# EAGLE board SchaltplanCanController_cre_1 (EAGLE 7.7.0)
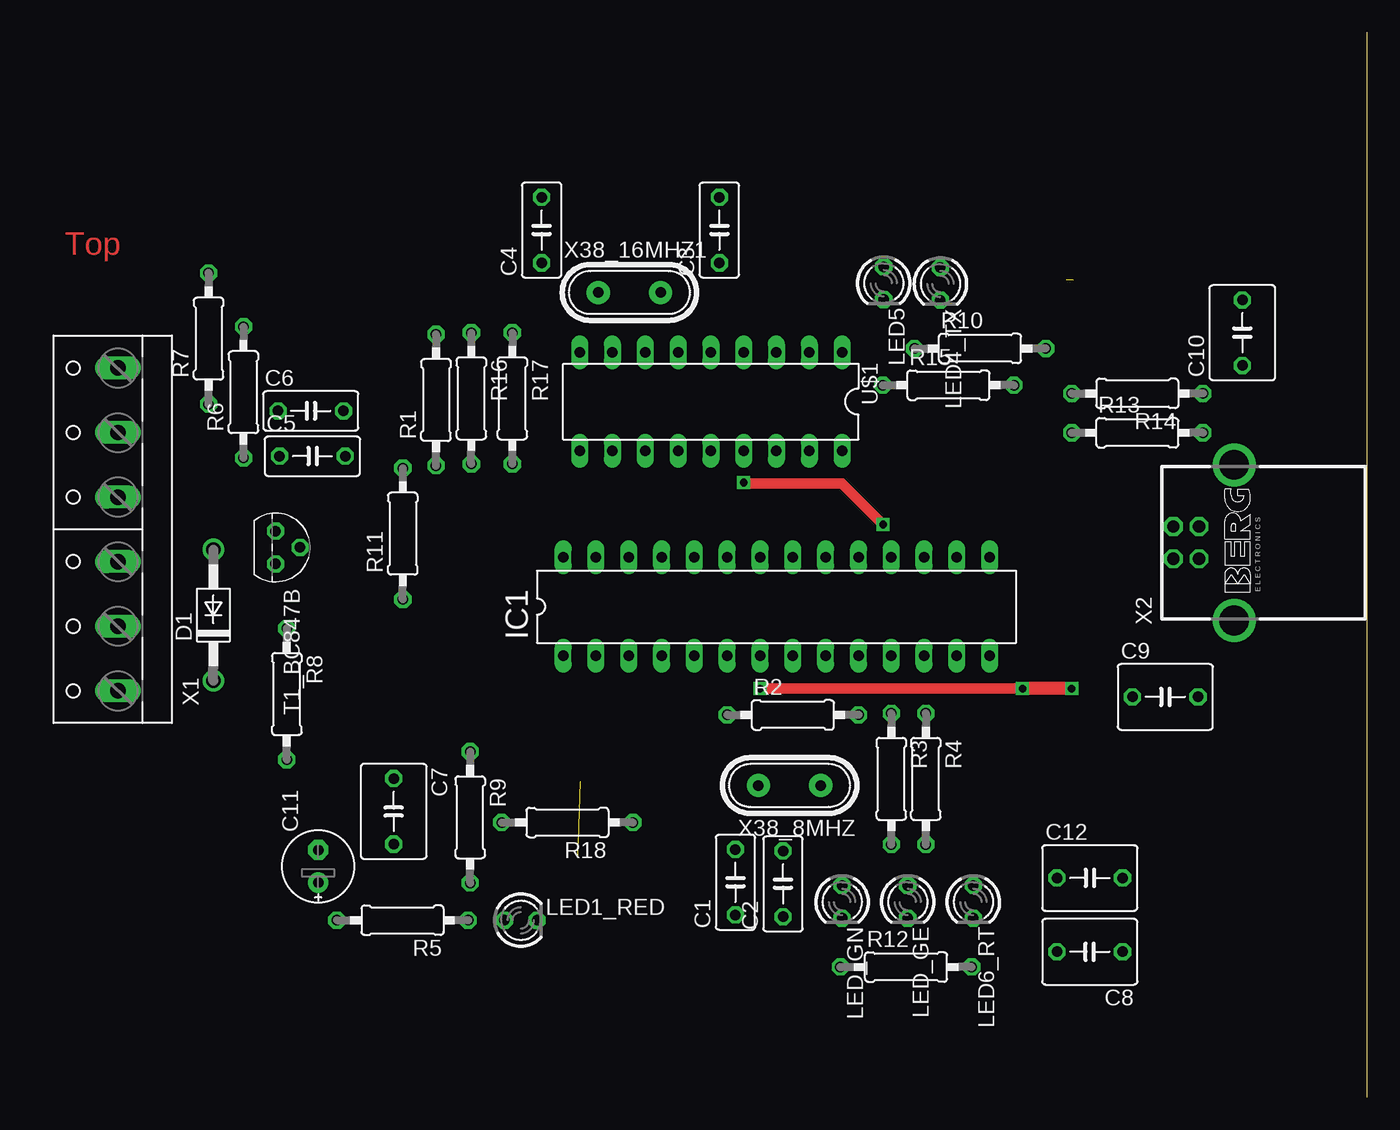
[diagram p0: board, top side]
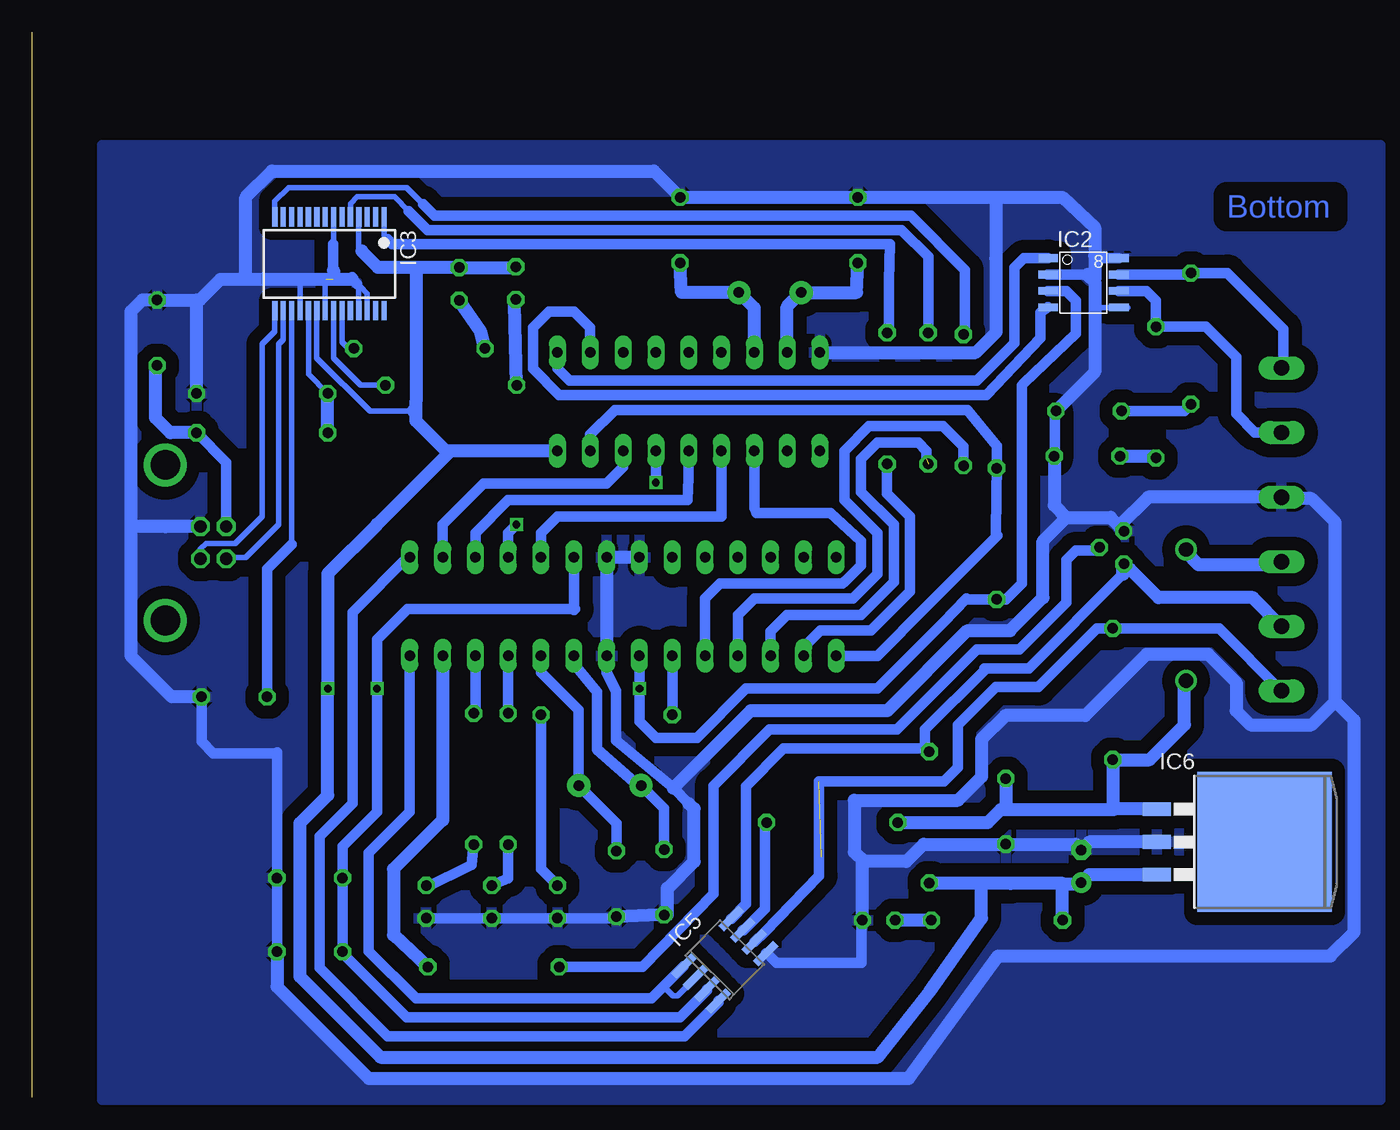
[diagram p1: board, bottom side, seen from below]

Size 0 x 82.46 mm. Coordinates in mm from the lower left corner, seen from the top.
Outline: 0,0 0,82.46
Copper layers (1*16): Top 0.035mm / dielectric 1.5mm / Bottom 0.035mm
Design rules "default": minimum track width 10mil, minimum drill 24mil, track to track 8mil, track to pad 8mil, pad to pad 8mil, via to via 8mil, smd to smd 8mil, copper to edge 40mil, drill to drill 8mil, minimum pad ring 10mil, minimum via ring 8mil, stop-mask expansion 4mil, vias tented up to drill 0mil, thermal gap 10mil

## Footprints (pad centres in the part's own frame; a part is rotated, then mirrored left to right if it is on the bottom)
C050-030X075 = drill 0.813 octagon: 1 -2.54,0; 2 2.54,0
C050-050X075 = drill 0.813 octagon: 1 -2.54,0; 2 2.54,0
E2,5-6E = drill 0.813 pad 1.575: + -1.27,0 | drill 0.813 pad 1.575 octagon: - 1.27,0
DO41-10 = drill 1.118: A 5.08,0; C -5.08,0
DIL28-3 = drill 0.813 long: 1 -16.51,-3.81; 2 -13.97,-3.81; 3 -11.43,-3.81; 4 -8.89,-3.81; 5 -6.35,-3.81; 6 -3.81,-3.81; 7 -1.27,-3.81; 8 1.27,-3.81; 9 3.81,-3.81; 10 6.35,-3.81; 11 8.89,-3.81; 12 11.43,-3.81; 13 13.97,-3.81; 14 16.51,-3.81; 15 16.51,3.81; 16 13.97,3.81; 17 11.43,3.81; 18 8.89,3.81; 19 6.35,3.81; 20 3.81,3.81; 21 1.27,3.81; 22 -1.27,3.81; 23 -3.81,3.81; 24 -6.35,3.81; 25 -8.89,3.81; 26 -11.43,3.81; 27 -13.97,3.81; 28 -16.51,3.81
DIL08 = smd 1.524 x 0.61: 1 -2.743,1.905; 2 -2.743,0.635; 3 -2.743,-0.635; 4 -2.743,-1.905; 5 2.743,-1.905; 6 2.743,-0.635; 7 2.743,0.635; 8 2.743,1.905
SSOP28 = smd 0.4 x 1.5: 1 -4.225,-3.625; 2 -3.575,-3.625; 3 -2.925,-3.625; 4 -2.275,-3.625; 5 -1.625,-3.625; 6 -0.975,-3.625; 7 -0.325,-3.625; 8 0.325,-3.625; 9 0.975,-3.625; 10 1.625,-3.625; 11 2.275,-3.625; 12 2.925,-3.625; 13 3.575,-3.625; 14 4.225,-3.625; 15 4.225,3.625; 16 3.575,3.625; 17 2.925,3.625; 18 2.275,3.625; 19 1.625,3.625; 20 0.975,3.625; 21 0.325,3.625; 22 -0.325,3.625; 23 -0.975,3.625; 24 -1.625,3.625; 25 -2.275,3.625; 26 -2.925,3.625; 27 -3.575,3.625; 28 -4.225,3.625
SO08 = smd 0.6 x 2.2: 1 -1.905,-2.6; 2 -0.635,-2.6; 3 0.635,-2.6; 4 1.905,-2.6; 5 1.905,2.6; 6 0.635,2.6; 7 -0.635,2.6; 8 -1.905,2.6
TO263-3 = smd 1.067 x 2.159: 1 -2.54,-5.791; 2 0,-5.791; 3 2.54,-5.791 | smd 10.8 x 10.41: TAB 0,2.54
LED3MM = drill 0.813 octagon: A -1.27,0; K 1.27,0
0207/10 = drill 0.813 octagon: 1 -5.08,0; 2 5.08,0
TO92 = drill 0.813 octagon: 1 1.27,0; 2 0,1.905; 3 -1.27,0
DIL18 = drill 0.813 long: 1 -10.16,-3.81; 2 -7.62,-3.81; 3 -5.08,-3.81; 4 -2.54,-3.81; 5 0,-3.81; 6 2.54,-3.81; 7 5.08,-3.81; 8 7.62,-3.81; 9 10.16,-3.81; 10 10.16,3.81; 11 7.62,3.81; 12 5.08,3.81; 13 2.54,3.81; 14 0,3.81; 15 -2.54,3.81; 16 -5.08,3.81; 17 -7.62,3.81; 18 -10.16,3.81
W237-6 = drill 1.194 long: 1 -12.5,-1.27; 2 -7.5,-1.27; 3 -2.5,-1.27; 4 2.5,-1.27; 5 7.5,-1.27; 6 12.5,-1.27
PN61729-S = drill 0.95 octagon: 1 1.25,4.71; 2 -1.25,4.71; 3 -1.25,2.71; 4 1.25,2.71 | drill 2.3 pad 2.9: S1 -6.02,0; S2 6.02,0
HC49 = drill 0.813 pad 1.8: 1 -2.413,0; 2 2.413,0

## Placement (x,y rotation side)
C1  22pF  [C050-030X075]  -48.91,16.65 90 top  (outside the outline)
C2  22pF  [C050-030X075]  -45.23,16.53 90 top  (outside the outline)
C3  22pF  [C050-030X075]  -50.16,67.15 90 top  (outside the outline)
C4  22pF  [C050-030X075]  -63.91,67.15 90 top  (outside the outline)
C5  560pF  [C050-030X075]  -81.66,49.64 0 top  (outside the outline)
C6  560pF  [C050-030X075]  -81.79,53.15 0 top  (outside the outline)
C7  100nF  [C050-050X075]  -75.37,22.14 270 top  (outside the outline)
C8  100nF  [C050-050X075]  -21.48,11.27 180 top  (outside the outline)
C9  100nF  [C050-050X075]  -15.64,31 0 top  (outside the outline)
C10  10nF  [C050-050X075]  -9.67,59.2 90 top  (outside the outline)
C11  10uf  [E2,5-6E]  -81.21,17.89 90 top  (outside the outline)
C12  100nF  [C050-050X075]  -21.48,16.98 0 top  (outside the outline)
D1  1N4004  [DO41-10]  -89.32,37.33 90 top  (outside the outline)
IC1  MEGA48/88/168-PU  [DIL28-3]  -45.73,37.99 0 top  (outside the outline)
IC2  SNOWND  [DIL08]  -81.38,63.07 0 bottom  (outside the outline)
IC3  FT232RL  [SSOP28]  -23,64.53 180 bottom  (outside the outline)
IC5  L9637D  [SO08]  -53.61,10.65 315 bottom  (outside the outline)
IC6  LM2937  [TO263-3]  -92.85,19.78 270 bottom  (outside the outline)
LED1_RED  2mA_+3,3V  [LED3MM]  -65.52,13.71 0 top  (outside the outline)
LED4_TX  2mA_TX  [LED3MM]  -33.04,62.98 270 top  (outside the outline)
LED5  2mA_RX  [LED3MM]  -37.43,63.03 270 top  (outside the outline)
LED6_RT  2mA mC  [LED3MM]  -30.49,15.13 270 top  (outside the outline)
LED_GE  2mA mC  [LED3MM]  -35.58,15.13 270 top  (outside the outline)
LED_GN  2mA mC  [LED3MM]  -40.65,15.13 270 top  (outside the outline)
R1  0  [0207/10]  -72.09,53.99 90 top  (outside the outline)
R2  270  [0207/10]  -44.46,29.61 0 top  (outside the outline)
R3  270  [0207/10]  -36.84,24.66 270 top  (outside the outline)
R4  270  [0207/10]  -34.18,24.66 270 top  (outside the outline)
R5  100  [0207/10]  -74.68,13.71 180 top  (outside the outline)
R6  100  [0207/10]  -87,54.59 90 top  (outside the outline)
R7  100  [0207/10]  -89.69,58.75 90 top  (outside the outline)
R8  510  [0207/10]  -83.64,31.22 270 top  (outside the outline)
R9  510  [0207/10]  -69.45,21.68 270 top  (outside the outline)
R10  270  [0207/10]  -29.97,57.98 0 top  (outside the outline)
R11  10k  [0207/10]  -74.66,43.64 90 top  (outside the outline)
R12  1k  [0207/10]  -35.7,10.09 0 top  (outside the outline)
R13  4k7  [0207/10]  -17.8,51.45 0 top  (outside the outline)
R14  10k  [0207/10]  -17.8,54.5 180 top  (outside the outline)
R15  270  [0207/10]  -32.42,55.13 0 top  (outside the outline)
R16  0  [0207/10]  -69.36,54.12 270 top  (outside the outline)
R17  0  [0207/10]  -66.18,54.12 270 top  (outside the outline)
R18  0  [0207/10]  -61.92,21.28 180 top  (outside the outline)
T1_BC847B  2N3565  [TO92]  -84.52,42.57 270 top  (outside the outline)
U$1  MCP2515DIL  [DIL18]  -50.81,53.87 180 top  (outside the outline)
X1  [W237-6]  -97.98,43.97 90 top  (outside the outline)
X2  PN61729-S  [PN61729-S]  -10.3,42.94 90 top  (outside the outline)
X38_8MHZ  CRYSTALS-NOGND-HC49  [HC49]  -44.72,24.15 180 top  (outside the outline)
X38_16MHZ1  CRYSTALS-NOGND-HC49  [HC49]  -57.12,62.31 0 top  (outside the outline)

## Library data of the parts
C1-C12 R1-R18 = rcl
D1 = diode
IC1 = avr-6
IC2 = SN65HVD231D
IC3 = ftdichip; MPN: FT232RL; OC_FARNELL: 1146032; OC_NEWARK: 91K9918
IC5 = st-microelectronics
IC6 = linear
LED1_RED LED4_TX LED5 LED6_RT LED_GE LED_GN = led
T1_BC847B = transistor
U$1 = MCP2515_MT
X1 = con-wago-500; OC_FARNELL: unknown; OC_NEWARK: unknown
X2 = con-berg; OC_FARNELL: unknown; OC_NEWARK: unknown
X38_8MHZ X38_16MHZ1 = IQD-Frequency-Products

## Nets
+5V: C8.2 C11.+ C12.1 IC1.7 IC1.20 IC2.3 IC3.4 IC3.20 IC5.3 IC6.3 LED4_TX.A LED5.A R5.2 R9.2 R11.1 U$1.18
+10V: C7.1 D1.C IC6.1 R8.2 R18.2
+12V: D1.A X1.3
GND: C1.1 C2.1 C3.2 C4.2 C5.2 C6.2 C7.2 C8.1 C9.2 C10.2 C11.- C12.2 IC1.8 IC1.21 IC1.22 IC2.2 IC2.8 IC3.7 IC3.18 IC3.21 IC3.25 IC3.26 IC5.5 IC6.2 LED1_RED.K LED6_RT.K LED_GE.K LED_GN.K R14.1 T1_BC847B.3 U$1.9 X1.4 X2.4
N$1: LED1_RED.A R5.1
N$2: IC1.1 R11.2 U$1.17
N$3: C1.2 IC1.9 X38_8MHZ.2
N$4: C5.1 R6.1
N$5: IC2.4 U$1.2
N$6: IC1.16 U$1.16
N$7: C2.2 IC1.10 X38_8MHZ.1
N$8: IC1.18 U$1.15
N$9: IC1.17 U$1.14
N$10: IC1.19 U$1.13
N$11: C3.1 U$1.7 X38_16MHZ1.2
N$12: C4.1 U$1.8 X38_16MHZ1.1
N$13: IC1.5 U$1.12
N$14: C6.1 R7.1
N$15: IC2.1 U$1.1
N$16: LED6_RT.A R4.2
N$17: IC1.14 IC5.1 IC5.2
N$18: IC1.15 IC5.4
N$19: IC3.16 X2.2
N$20: IC2.6 R6.2 X1.5
N$21: IC2.7 R7.2 X1.6
N$23: LED5.K R15.1
N$24: LED_GN.A R2.2
N$25: IC1.6 R2.1
N$26: IC1.11 R3.1
N$27: IC1.12 R4.1
N$28: LED_GE.A R3.2
N$29: IC3.15 X2.3
N$30: LED4_TX.K R10.1
N$31: IC1.2 R17.2
N$32: IC3.22 R15.2
N$33: IC5.6 R8.1 X1.1
N$34: R12.1 T1_BC847B.2
N$35: IC1.13 R12.2
N$36: IC5.8 R9.1 T1_BC847B.1 X1.2
N$37: C10.1 R13.2 X2.1
N$38: C9.1 IC3.17
N$39: IC3.23 R10.2
N$40: IC3.14 R1.2
N$41: IC1.4 R1.1
N$42: IC3.1 R17.1
N$43: IC5.7 R18.1
N$45: IC1.3 R16.2
N$46: IC3.5 R16.1
N$47: IC3.19 R13.1 R14.2

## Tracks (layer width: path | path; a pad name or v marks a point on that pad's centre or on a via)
+5V  (via drill 0.6)
  Top 0.813: v-47,31.64 v-26.69,31.64
  Top 1.016: v-22.88,31.64 v-26.69,31.64
  Bottom 0.406: IC3.4 -25.28,65.56 -25.5,65.52 | IC3.20 -22.03,57.25 -26.14,53.13 -29.51,53.13 -29.69,53.87
  Bottom 0.813: IC1.20 -41.92,37.72 -42.02,37.81 -29.05,37.81 -26.69,35.45 v-26.69,31.64 -26.69,22.11 -24.02,19.45 C12.1 C8.2 -24.02,11.15 -28.96,6.21 -50.13,6.21 -52.22,8.29 IC5.3 | IC1.7 v-47,31.64 -47,29.1 -48.27,27.83 -51.45,27.83 -55.26,31.64 -65.42,31.64 -70.5,36.72 -72.32,38.62 -72.39,38.56 R11.1 -75.37,38.56 -76.6,39.78 -76.6,55.12 -76.78,55.3 -80.79,59.13 -80.79,61.69 -80.04,62.44 IC2.3
  Bottom 1.016: U$1.18 -32.4,50.05 | -32.4,50.05 -26.69,44.34 -26.69,44.36 -22.88,40.55 v-22.88,31.64 -22.88,23.39 -20.7,21.21 -20.7,9.36 -26.96,3.1 -65.47,3.1 -69.48,8.21 -73.5,13.87 -73.5,16.6 | R9.2 -73.5,16.6 | -73.5,16.6 -75.69,16.6 | -75.69,16.6 -79.7,16.6 -79.76,16.54 | -75.75,16.54 -75.69,16.6 | R5.2 -79.76,16.54 | IC6.3 -81.83,17.24 C11.+ -81.13,16.54 -79.76,16.54 | LED5.A -37.01,64.25 LED4_TX.A -29.7,64.25 | -29.7,64.25 -29.69,64.24 -29.69,53.87 | -32.4,50.05 -32.02,50.05 -29.69,52.38 -29.69,53.68 -29.51,53.13 | -29.7,64.25 -26.77,64.25 -25.5,65.52
+10V
  Bottom 1.016: -83.72,22.27 -83.64,22.34 R8.2 -86.5,26.14 -89.19,28.84 -89.19,32.12 D1.C | IC6.1 -83.77,22.32 -83.72,22.27 | -83.72,22.27 -75.32,22.27 | -75.32,22.27 -74.95,22.27 -73.97,21.29 R18.2 | C7.1 -75.37,22.32 -75.32,22.27
+12V
  Bottom 1.016: D1.A -89.32,42.2 -90.28,41.24 -96.48,41.24 X1.3
GND  (1 unrouted)
  Bottom 0.406: IC3.25 -25.28,62.62 -25.41,62.76 | IC3.21 -22.68,63.24 -22.76,63.33 | IC3.18 -20.73,63.3 -20.75,63.33 | IC3.26 -25.93,62.24 -25.41,62.76 | -25.41,62.76 -25.34,62.76 -25.13,62.96 | IC3.7 -23.33,64.04 -23.49,63.88
  Bottom 0.813: LED6_RT.K LED_GE.K LED_GN.K -45.1,13.86 C2.1 | IC1.8 -44.46,32.91 -45.19,31.46 -45.19,27.65 -49.62,23.94 -50.81,22.75 | C1.1 -49.16,14.11 | C8.1 C12.2 -18.94,26.69 -18.9,26.64 -14,26.64 -13.1,27.55 C9.2 | IC2.2 -81.69,63.71 -82.25,63.33 | IC5.5 -56.88,11.14 -57.62,10.4 -64.19,10.4 -64.19,13.65 LED1_RED.K | IC2.8 -82.43,64.98 -82.25,65.15 | -24.77,63.51 -24.77,63.33 -25.13,62.96
  Bottom 1.016: C1.1 -48.53,14.11 C2.1 | U$1.9 -73.04,57.67 -74.63,59.26 -74.63,64.93 | IC1.22 IC1.21 IC1.8 | -10.32,44.19 X2.4 -7.78,44.19 -7.63,44.34 | R14.1 -12.71,61.74 | -12.71,61.74 C10.2 -8.52,61.74 -7.63,60.85 -7.63,44.34 | -12.71,61.74 -12.97,61.74 -14.56,63.33 -16.52,63.33 | -7.63,44.34 -7.63,34.18 -10.81,31 C9.2 | -49.62,23.94 -55.61,29.93 -66.19,29.93 -72.4,36.13 -75.69,36.13 -78.24,38.69 -78.24,43.07 -80.06,44.9 | -49.16,14.11 -49.16,16.18 -51.23,18.25 -51.23,22.34 -50.81,22.75 | -80.06,44.9 -83.46,44.9 -84.14,44.22 | -84.14,44.22 T1_BC847B.3 | X1.4 -96.12,46.47 | -96.12,46.47 -86.38,46.47 -84.14,44.22 | -64.37,18.25 -67.66,18.25 -69.01,19.6 C7.2 -80.77,19.6 C11.- -81.83,19.78 IC6.2 | LED1_RED.K -64.25,18.13 -64.37,18.25 | -64.37,18.25 -63.64,18.98 -63.64,23 -71.67,23 -73.5,24.82 -73.5,27.74 -75.32,29.57 -81.52,29.57 -86.27,34.31 -91.02,34.31 -93.2,32.12 -93.2,29.93 -94.3,28.84 -99.05,28.84 -100.87,30.66 | -100.87,30.66 -100.87,44.53 -99.05,46.35 -96.24,46.35 -96.12,46.47 | C8.1 -18.94,8.57 -26.05,1.46 -67.84,1.46 -74.77,10.95 -100.5,10.95 -102.33,12.78 -102.33,29.2 -100.87,30.66 | C5.2 -79.12,45.84 -80.06,44.9 | -82.25,63.33 -82.25,65.15 -82.25,67.34 -79.73,69.69 -74.41,69.69 | -81.69,63.71 -82.25,63.15 -82.25,56.16 C6.2 | -74.63,64.93 -74.59,64.97 | -74.41,69.69 C4.2 C3.2 -48.12,71.72 -18.56,71.72 -16.52,69.69 -16.52,63.33 | -74.63,64.93 -74.63,69.47 -74.41,69.69 | -24.77,63.33 -23.31,63.33 | -23.31,63.33 -20.75,63.33 -16.52,63.33 | -23.33,64.04 -23.33,63.35 -23.31,63.33
  pour Bottom (isolate 1.016): -5.42,-0.18 -5.42,73.73 -104.34,73.73 -104.34,-0.18
N$1
  Bottom 1.016: R5.1 LED1_RED.A
N$2
  Bottom 0.813: U$1.17 -43.19,51.33 -45.1,53.23 -72.41,53.23 -74.66,50.43 R11.2 -74.64,46.88 -74.6,43.41 -74.7,43.52 -69.23,37.99 -65.42,34.18 IC1.1
N$3
  Bottom 0.813: C1.2 -48.91,22.37 X38_8MHZ.2 -46.88,24.15 -43.73,26.93 -43.73,31.37 -41.92,33.55 IC1.9
N$4
  Bottom 1.016: C5.1 -86.86,49.64 R6.1
N$5
  Bottom 0.813: U$1.2 -43.19,59.58 -41.92,60.85 -40.02,60.85 -38.75,59.58 -38.75,56.41 -40.77,54.38 -73.86,54.38 -78.06,58.77 -78.06,60.77 IC2.4
N$6
  Bottom 0.813: U$1.16 -45.73,48.78 -44.46,47.52 -34.94,47.52 -31.77,44.34 IC1.16
N$7
  Bottom 0.813: C2.2 -45.23,21.23 X38_8MHZ.1 -42.31,29.99 -39.38,32.91 IC1.10
N$8  (via drill 0.6)
  Top 0.813: v-37.48,44.34 -40.65,47.52 -47.64,47.52 v-48.27,47.6
  Bottom 0.813: IC1.18 -36.84,43.7 v-37.48,44.34 | v-48.27,47.6 U$1.15
N$9
  Bottom 0.813: U$1.14 -50.81,47.97 -50.73,46.24 -36.84,46.24 -34.3,43.7 IC1.17
N$10
  Bottom 0.813: U$1.13 -53.35,47.52 -53.37,44.98 -40.65,44.98 -39.38,43.7 IC1.19
N$11
  Bottom 1.016: U$1.7 -55.89,61.12 X38_16MHZ1.2 -50.26,62.31 C3.1
N$12
  Bottom 1.016: U$1.8 -58.43,61.22 X38_16MHZ1.1 -63.8,62.31 C4.1
N$13
  Bottom 0.813: U$1.12 -55.89,45.61 -56.07,45.25 -61.78,45.25 -64.15,43.07 -64.15,41.16 -62.88,39.9 -62.84,39.9 -62.73,39.78 -53.24,39.78 -52.08,38.62 IC1.5
N$14
  Bottom 0.813: C6.1 -89.18,53.15 R7.1
N$15
  Bottom 0.813: U$1.1 -40.65,56.41 -41.58,55.48 -73.13,55.48 -76.05,58.4 -76.05,64.24 -76.78,64.97 IC2.1
N$16
  Bottom 0.813: R4.2 -33.99,18 -30.39,16.22 LED6_RT.A
N$17
  Bottom 0.406: IC5.2 -51.32,9.22 -49.95,7.85 -49.59,7.85 -48.86,8.58
  Bottom 0.813: IC1.14 -29.22,22.11 -26.05,18.93 -26.05,11.31 -29.69,7.67 -47.94,7.67 -48.86,8.58 -50.42,10.14 IC5.1
N$18
  Bottom 0.813: IC1.15 -29.22,41.99 -24.78,37.55 -24.78,22.75 -22.24,20.21 -22.24,10.01 -27.5,4.75 -50.5,4.75 -53.12,7.36 IC5.4
N$19
  Bottom 0.406: IC3.16 -19.43,58.67 -19.06,58.31 -19.06,44.34 -16.52,41.8 -15.12,41.8 X2.2
N$20
  Bottom 0.813: X1.5 -94.66,51.47 -93.2,52.92 -93.2,57.3 -90.84,59.67 R6.2 -87,61.69 -86.25,62.44 IC2.6
N$21
  Bottom 0.813: X1.6 -96.85,56.62 -96.85,59.49 -92.52,63.83 R7.2 -89.57,63.71 IC2.7
N$23
  Bottom 1.016: R15.1 -37.32,61.47 LED5.K
N$24
  Bottom 0.813: R2.2 -39.38,17.67 LED_GN.A
N$25
  Bottom 0.813: IC1.6 R2.1
N$26
  Bottom 0.813: R3.1 IC1.11
N$27
  Bottom 0.813: IC1.12 -34.3,29.86 R4.1
N$28
  Bottom 0.813: R3.2 -36.84,16.94 LED_GE.A
N$29
  Bottom 0.406: X2.3 -13.01,42.45 -13.45,42.89 -15.71,42.89 -17.8,44.98 -17.8,58.31 -18.78,59.29 IC3.15
N$30
  Bottom 1.016: R10.1 -34.69,59.34 LED4_TX.K
N$31
  Bottom 0.813: R17.2 -66.18,46.75 -67.96,44.98 -67.96,39.18 -64.92,36.13 -61.02,36.13 -59.7,34.81 IC1.2
N$32
  Bottom 0.406: IC3.22 -23.33,57.22 -25.41,55.13 R15.2
N$33  (1 unrouted)
  Bottom 0.813: X1.1 -91.88,36.3 R8.1 -82.42,36.3 -77.88,31.75 -74.59,31.75 -71.67,28.84 -71.67,25.55 -70.57,24.45 -61.08,24.45 | -60.9,24.45 -61.08,24.45 | IC5.6 -56.7,12.77 -60.9,17.16 -60.9,24.27 -61.08,24.45
N$34
  Bottom 0.813: R12.1 -47.23,10.09 -52.72,15.77 -52.72,24.12 -57.07,28.47 -66.92,28.47 -73.13,34.67 -76.41,34.67 -80.06,38.33 -80.06,41.61 -80.79,42.34 -82.38,42.34 T1_BC847B.2
  Bottom 1.016: T1_BC847B.2
N$35
  Bottom 1.016: IC1.13 -31.77,21.48 -27.95,17.67 -27.95,12.57 R12.2
N$36
  Bottom 0.813: -84.44,40.52 -77.14,33.22 -73.71,33.22 -73.71,33.07 -69.11,28.47 -69.11,27.1 R9.1 -69.2,27.01 -58.16,27.01 -55.24,24.09 -55.24,14.96 -54.11,13.83 IC5.8
  Bottom 1.016: X1.2 -94.49,38.69 -87.18,38.69 -84.99,40.88 -84.94,40.88 T1_BC847B.1 -84.44,41.23 -84.44,40.52
N$37
  Bottom 0.813: X2.1 -15.01,49.16 R13.2
  Bottom 1.016: R13.2 -10.68,51.45 -9.54,52.59 -9.54,56.53 C10.1
N$38
  Bottom 0.406: IC3.17 -20.08,42.81
  Bottom 0.813: C9.1 -18.18,40.91 -20.08,42.81
N$39
  Bottom 0.406: R10.2 -24.53,57.93 -23.98,58.48 IC3.23
N$40
  Bottom 0.406: IC3.14 -18.78,69.38 -19.84,70.44 -28.96,70.44 -30.24,69.17 -30.61,68.8
  Bottom 0.813: -72.09,59.26 R1.2 -72.22,59.2 -72.22,64.06 -68.02,68.25 -31.16,68.25 -30.24,69.17
N$41
  Bottom 0.813: IC1.4 -54.62,37.35 -55.89,38.62 -63.51,38.62 -65.42,40.53 -65.42,43.7 -62.88,46.24 -62.88,50.05 -64.78,51.96 -70.5,51.96 -72.09,50.37 R1.1
N$42
  Bottom 0.406: IC3.1 -27.23,66.71 -27.5,66.43
  Bottom 0.813: R17.1 -66.31,59.2 -66.32,60.3 -66.32,63.2 -66.38,66.06 -27.87,66.06 -27.5,66.43
N$43
  Bottom 0.813: IC5.7 -55.04,12.94 -56.7,14.6 -56.7,21.14 R18.1
N$45  (1 unrouted)
  Bottom 0.813: IC1.3 -57.16,36.09 -58.43,37.35 -64.15,37.35 -66.69,39.9 -66.69,44.34 -64.15,46.88 -64.15,49.42 -65.42,50.69 -68.59,50.69 -69.23,50.05 -69.23,49.42
N$46
  Bottom 0.406: IC3.5 -24.63,69.21 -25.13,69.72 -28.05,69.72 -29.15,68.62
  Bottom 0.813: R16.1 -69.36,65.09 -67.29,67.16 -30.61,67.16 -29.15,68.62
N$47
  Bottom 0.406: IC3.19 -21.38,56 R14.2
  Bottom 1.016: R13.1 R14.2
S$1
  Bottom 0.406: -82.07,61.14 -84.26,61.14 -84.81,61.14
S$3
  Bottom 0.813: -79.15,53.11 -79.15,49.46
S$4
  Bottom 0.813: -23.31,63.69 -23.31,66.06

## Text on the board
Top: Top
Bottom: Bottom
